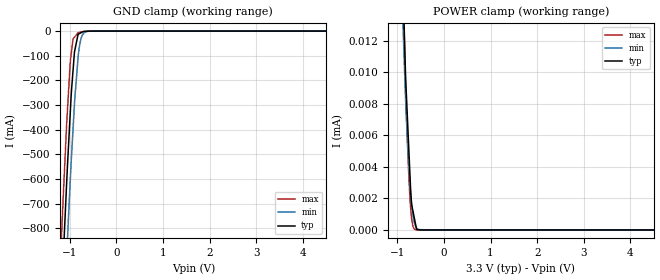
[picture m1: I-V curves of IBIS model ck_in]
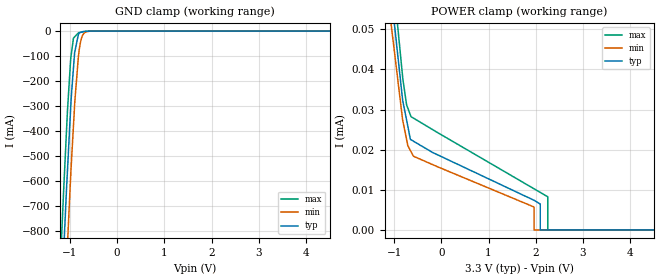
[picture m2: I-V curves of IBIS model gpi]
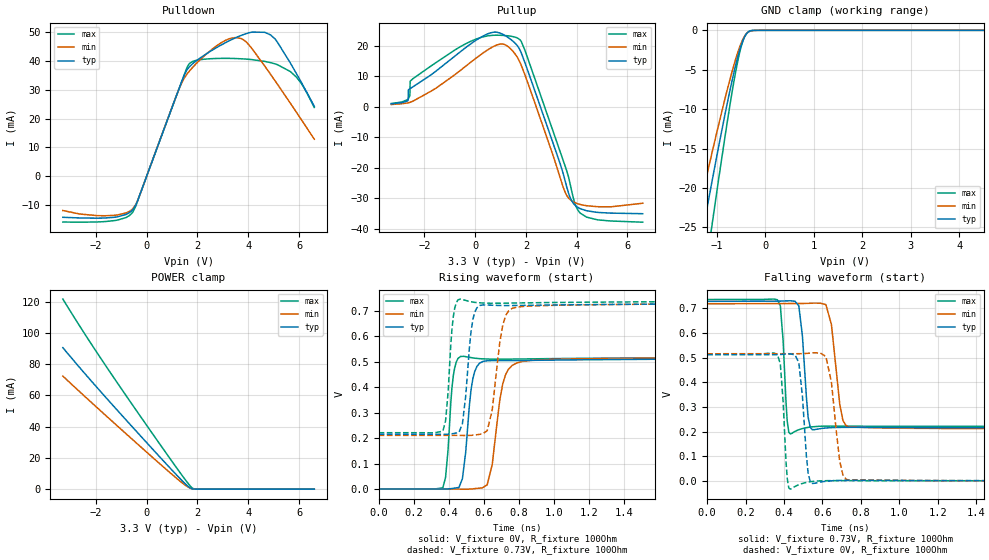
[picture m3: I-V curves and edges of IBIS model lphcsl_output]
|Texas Instruments Incorporated
| Marketing Part # : CDCDB2000
| Voltage Range : 3.3V
| Package-type: TLGA (GQFN)
| #pins/pkg drawing : 80-pin NPP
[IBIS Ver] 3.2
[File name] cdcdb2000.ibs
[File Rev] 1.1
[Date] 04/19/2023
[Source]
| Texas Instruments Incorporated.
| 12500 TI Blvd
| Dallas, TX -75243
[Notes] Revision History:
| Rev 1.1: 04/19/2023
| - Output model updated to take into account impedance values
| - after production trim
| Rev 1.0: 02/18/2019
| - Initial version of the model
| - Model generated from simulations in TISPICE/SPECTRE
| - C_comp although listed in numerical order of value are
| obtained from varying PVT conditions. For PVT conditions for
| each specific value refer the buffer description under
| respective [Model]. IBIS model user is responsible for using
| appropriate C_comp to simulate for Signal Integrity.
| - Warnings regarding combined Non-monotonicity of various models have been
| reviewed and considered minor and can be ignored.
|**** Modify the following if you use [Model Selector]*****************
| - Model names with a trailing _1p8 contain the model for
| 1.8V operation. Model names with a trailing _3p3 contain the model
| for 3.3V operation.
[Disclaimer]
| This model is designed as an aid for customers of Texas Instruments.
| TI and its licensors and suppliers make no warranties, either expressed
| or implied, with respect to this model, including the warranties of
| merchantability or fitness for a particular purpose. The model is
| provided solely on an "as is" basis. The entire risk as to its quality
| and performance is with the customer.
| This model is subject to change without notice. Texas Instruments
| Incorporated is not responsible for updating this model.
[Copyright]
(C) Copyright 2019 Texas Instruments Incorporated. All rights reserved.
| Component1 CDCDB2000 (per package)
[Component] CDCDB2000
[Manufacturer] Texas Instruments Incorporated
[Package] |80 GQFN
| variable typ min max
R_pkg 0.111 0.052 0.169
L_pkg 2.02nH 1.12nH 2.9nH
C_pkg 0.163pF 0.062pF 0.264pF
| pin number (pin name) mapping to model name
[Pin] signal_name model_name R_pin L_pin C_pin
1   DIF_INP   ck_in   NA   NA   NA
2   DIF_INN   ck_in   NA   NA   NA
3   DIF0P   lphcsl_output   NA   NA   NA
4   DIF0N   lphcsl_output   NA   NA   NA
5   DIF1P   lphcsl_output   NA   NA   NA
6   DIF1N   lphcsl_output   NA   NA   NA
7   DIF2P   lphcsl_output   NA   NA   NA
8   DIF2N   lphcsl_output   NA   NA   NA
9   DIF3P   lphcsl_output   NA   NA   NA
10   DIF3N   lphcsl_output   NA   NA   NA
11   DIF4P   lphcsl_output   NA   NA   NA
12   DIF4N   lphcsl_output   NA   NA   NA
13   DIF5P   lphcsl_output   NA   NA   NA
14   DIF5N   lphcsl_output   NA   NA   NA
15   DIF6P   lphcsl_output   NA   NA   NA
16   DIF6N   lphcsl_output   NA   NA   NA
17   DIF7P   lphcsl_output   NA   NA   NA
18   DIF7N   lphcsl_output   NA   NA   NA
19   DIF8P   lphcsl_output   NA   NA   NA
20   DIF8N   lphcsl_output   NA   NA   NA
21   DIF9P   lphcsl_output   NA   NA   NA
22   DIF9N   lphcsl_output   NA   NA   NA
23   DIF10P   lphcsl_output   NA   NA   NA
24   DIF10N   lphcsl_output   NA   NA   NA
25   DIF11P   lphcsl_output   NA   NA   NA
26   DIF11N   lphcsl_output   NA   NA   NA
27   DIF12P   lphcsl_output   NA   NA   NA
28   DIF12N   lphcsl_output   NA   NA   NA
29   DIF13P   lphcsl_output   NA   NA   NA
30   DIF13N   lphcsl_output   NA   NA   NA
31   DIF14P   lphcsl_output   NA   NA   NA
32   DIF14N   lphcsl_output   NA   NA   NA
33   DIF15P   lphcsl_output   NA   NA   NA
34   DIF15N   lphcsl_output   NA   NA   NA
35   DIF16P   lphcsl_output   NA   NA   NA
36   DIF16N   lphcsl_output   NA   NA   NA
37   DIF17P   lphcsl_output   NA   NA   NA
38   DIF17N   lphcsl_output   NA   NA   NA
39   DIF18P   lphcsl_output   NA   NA   NA
40   DIF18N   lphcsl_output   NA   NA   NA
41   DIF19P   lphcsl_output   NA   NA   NA
42   DIF19N   lphcsl_output   NA   NA   NA
43   POWERGD   gpi   NA   NA   NA
44   OE5B/DATA   gpi   NA   NA   NA
45   OE6B/CLK   gpi   NA   NA   NA
46   OE7B   gpi   NA   NA   NA
47   OE8B   gpi   NA   NA   NA
48   OE9B   gpi   NA   NA   NA
49   OE10B/SHIFT_LD   gpi   NA   NA   NA
50   OE11B   gpi   NA   NA   NA
51   OE12B   gpi   NA   NA   NA
52   SADR0   strap_in   NA   NA   NA
53   SADR1   strap_in   NA   NA   NA
54   VDD   POWER   NA   NA   NA
55   SBEN   gpi   NA   NA   NA
56   VDD_A   POWER   NA   NA   NA
57   SMBDAT   smbdat   NA   NA   NA
58   SMBCLK   smbclk   NA   NA   NA
[Diff Pin]   inv_pin   vdiff   tdelay_typ  tdelay_min  tdelay_max
1   2   10m   NA   NA   NA
3   4   NA   NA   NA   NA
5   6   NA   NA   NA   NA
7   8   NA   NA   NA   NA
9   10   NA   NA   NA   NA
11   12   NA   NA   NA   NA
13   14   NA   NA   NA   NA
15   16   NA   NA   NA   NA
17   18   NA   NA   NA   NA
19   20   NA   NA   NA   NA
21   22   NA   NA   NA   NA
23   24   NA   NA   NA   NA
25   26   NA   NA   NA   NA
27   28   NA   NA   NA   NA
29   30   NA   NA   NA   NA
31   32   NA   NA   NA   NA
33   34   NA   NA   NA   NA
35   36   NA   NA   NA   NA
37   38   NA   NA   NA   NA
39   40   NA   NA   NA   NA
41   42   NA   NA   NA   NA
| Use Differential pin definition for differential I/Os
|[Diff Pin] inv_pin vdiff tdelay_typ tdelay_min tdelay_max
|3 4 200mV NA NA NA
|15 16 NA NA NA NA
|***** end of component 1 definition
| Models and submodels in the file (6): ck_in (Input), gpi (Input), lphcsl_output (Output), smbclk (Input), smbdat (I/O_open_drain), strap_in (Input)
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| Model Selectors
|***Modify the following as it applies to a speciic model with multiple ****
|*** powver supply options or driver programmability *********
| Model1
|IBIS Model File - Generated by SIMDE
| http://www.iometh.com/Product/SIMDE
[Model]   ck_in
Model_type   Input
Vinl = 0.66
Vinh = 2.64
|   typ   min   max
C_comp   1.16pF   1.09pF   1.19pF
[Voltage Range]   3.3   3.135   3.465
[Temperature Range]   27   105   -40
[Power Clamp Reference]   3.3   3.135   3.465
[GND Clamp Reference]   0   0   0
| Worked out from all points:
|   GND clamp passes 1 mA (typ) near -0.66 V on its own axis
|   POWER clamp passes 1 mA (typ) near -3.28 V on its own axis
[GND Clamp]
|   Voltage   I(typ)   I(min)   I(max)
-3.3V     -11.22A    -11.44A    -11.05A
-1.173V   -1.062A    -1.366A    -813.7mA
-1.136V   -902.5mA   -1.208A    -656.9mA
-1.079V   -664.6mA   -960.5mA   -423.2mA
-1.053V   -557.2mA   -856mA     -329.6mA
-983.9mV  -310.7mA   -583.3mA   -113.4mA
-930.4mV  -160.9mA   -399.1mA   -32.16mA
-899.2mV  -84.55mA   -294.1mA   -24.93mA
-819.1mV  -12.84mA   -100.7mA   -6.285mA
-733.2mV  -4.01mA    -17.71mA   -3.143mA
-574.9mV  -160.4uA   -530.3uA   -296uA
6.6V      0A         0A         0A
[POWER Clamp]
|   Voltage   I(typ)   I(min)   I(max)
-3.3V     1.02mA     538.7uA    1.487mA
-1.308V   59.88uA    49.8uA     64.78uA
-821.7mV  9.697uA    8.259uA    8.987uA
-767.8mV  6.116uA    4.856uA    4.476uA
-742.7mV  4.452uA    3.567uA    2.814uA
-721.9mV  3.073uA    2.634uA    1.725uA
-711.4mV  2.376uA    2.259uA    1.354uA
-693.3mV  1.637uA    1.625uA    731nA
-636.6mV  790nA      481.6nA    47.81nA
-586.5mV  40.89nA    122.5nA    5.344nA
-503.6mV  0A         20.62nA    0A
6.6V      0A         0A         0A
[Model]   gpi
Model_type   Input
Vinl = 1.2
Vinh = 1.6
|   typ   min   max
C_comp   0.852pF   0.823pF   0.899pF
[Voltage Range]   3.3   3.135   3.465
[Temperature Range]   27   105   -40
[Power Clamp Reference]   3.3   3.135   3.465
[GND Clamp Reference]   0   0   0
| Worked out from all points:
|   GND clamp passes 1 mA (typ) near -0.67 V on its own axis
|   POWER clamp passes 1 mA (typ) near -3.23 V on its own axis
[GND Clamp]
|   Voltage   I(typ)   I(min)   I(max)
-3.3V     -11.22A    -11.44A    -11.05A
-1.169V   -1.043A    -1.347A    -794.9mA
-1.117V   -822.5mA   -1.123A    -578.3mA
-1.052V   -561.1mA   -858mA     -321.1mA
-981.8mV  -301.3mA   -575.6mA   -108.9mA
-924.3mV  -147.1mA   -378.9mA   -28.07mA
-900.2mV  -86.41mA   -297.7mA   -23.27mA
-814.3mV  -11.35mA   -92.89mA   -6.206mA
-776.1mV  -5.231mA   -44.91mA   -4.896mA
-733.4mV  -2.522mA   -17.99mA   -3.434mA
-576.2mV  -234.6uA   -567.7uA   -301.8uA
6.6V      0A         0A         0A
[POWER Clamp]
|   Voltage   I(typ)   I(min)   I(max)
-3.3V     1.056mA    570.2uA    1.534mA
-1.562V   113.2uA    100.1uA    127.7uA
-818.6mV  32.32uA    27.41uA    38.13uA
-594.1mV  22.15uA    18.47uA    27.9uA
1.964V    7.396uA    5.719uA    10.26uA
1.965V    7.392uA    5.625uA    10.26uA
1.965V    7.392uA    0A         10.26uA
2.096V    0A         0A         9.361uA
2.255V    0A         0A         8.268uA
2.255V    0A         0A         8.026uA
2.255V    0A         0A         0A
6.6V      0A         0A         0A
[Model]   lphcsl_output
Model_type   Output
Polarity   Non-Inverting
Vmeas = 0.375
Vref = 0.375
Cref = 2pF
Rref = 100000
|   typ   min   max
C_comp   0.625pF   0.558pF   0.773pF
[Voltage Range]   3.3   3.135   3.465
[Temperature Range]   27   125   -40
[Pullup Reference]   3.3   3.135   3.465
[Pulldown Reference]   -0   -0   -0
[Power Clamp Reference]   3.3   3.135   3.465
[GND Clamp Reference]   0   0   0
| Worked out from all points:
|   slope of the pulldown table from 0 to 0.495 V, typ, clamps not added: 41.7 ohm
|   GND clamp passes 1 mA (typ) near -0.44 V on its own axis
|   falling waveform, V_fixture 0.73V, R_fixture 100Ohm: 20-80 % time 29ps typ, 40.6ps min, 21.3ps max; typ from 0.728 V to 0.215 V
|   rising waveform, V_fixture 0V, R_fixture 100Ohm: 20-80 % time 42.6ps typ, 58.6ps min, 31.4ps max; typ from 0 V to 0.51 V
|   rising waveform, V_fixture 0.73V, R_fixture 100Ohm: 20-80 % time 40ps typ, 54.5ps min, 30.1ps max; typ from 0.215 V to 0.727 V
|   falling waveform, V_fixture 0V, R_fixture 100Ohm: 20-80 % time 29.6ps typ, 43ps min, 22.1ps max; typ from 0.512 V to 0.001 V
[Pulldown]
|   Voltage   I(typ)   I(min)   I(max)
-3.3V     -14.26mA   -11.91mA   -15.9mA
-1.637V   -14.51mA   -13.73mA   -15.74mA
-547.8mV  -11.64mA   -11.28mA   -12.45mA
-260.7mV  -6.256mA   -6.291mA   -6.246mA
1.264V    30.12mA    30.06mA    30.14mA
1.67V     37.85mA    36.36mA    38.96mA
2.65V     44.12mA    44.59mA    40.85mA
3.343V    47.42mA    47.95mA    40.9mA
3.897V    49.43mA    46.82mA    40.67mA
4.877V    49.05mA    35.38mA    39.43mA
5.887V    35.76mA    22.33mA    34.47mA
6.6V      24.26mA    12.85mA    23.87mA
[GND Clamp]
|   Voltage   I(typ)   I(min)   I(max)
-3.3V     -95.21mA   -78.35mA   -123.7mA
-1.538V   -33.84mA   -27.44mA   -43.92mA
-1.34V    -27.13mA   -21.99mA   -35.15mA
-1.241V   -23.81mA   -19.3mA    -30.8mA
-1.112V   -19.56mA   -15.85mA   -25.22mA
-1.003V   -16.02mA   -12.99mA   -20.56mA
-815.1mV  -10.12mA   -8.246mA   -12.78mA
-587.4mV  -3.811mA   -3.16mA    -4.469mA
-458.7mV  -1.229mA   -1.073mA   -1.272mA
-389.4mV  -433.8uA   -414.9uA   -415uA
-320.1mV  -93.44uA   -113.8uA   -78.75uA
6.6V      0A         0A         0A
[Pullup]
|   Voltage   I(typ)   I(min)   I(max)
-3.3V     954.3uA    732.8uA    1.056mA
-2.637V   2.12mA     1.291mA    2.559mA
-2.627V   5.549mA    1.309mA    2.656mA
-2.567V   5.892mA    1.44mA     3.69mA
-2.558V   5.947mA    1.466mA    8.374mA
-2.449V   6.527mA    1.821mA    9.191mA
432.3mV   23.67mA    18.3mA     23.14mA
1.125V    23.59mA    20.53mA    23.38mA
1.68V     19.83mA    15.99mA    22.47mA
3.551V    -24.51mA   -28.15mA   -19.62mA
4.046V    -33.01mA   -31.84mA   -33.9mA
6.6V      -35.08mA   -31.64mA   -37.86mA
[POWER Clamp]
|   Voltage   I(typ)   I(min)   I(max)
-3.3V     90.61mA    72.41mA    121.7mA
-2.162V   68.92mA    55.3mA     92.49mA
-815.1mV  44.38mA    35.53mA    60mA
1.214V    8.474mA    6.479mA    12.85mA
1.61V     2.102mA    1.548mA    4.142mA
1.798V    256.2uA    261uA      767.7uA
1.967V    5.611uA    12.37uA    12.29uA
6.6V      0A         0A         0A
[Ramp]
R_load = 100
|   typ   min   max
dV/dt_r   0.305979/4.26211e-11   0.308993/5.85849e-11   0.309345/3.13767e-11
dV/dt_f   0.307804/2.8961e-11   0.30405/4.06149e-11   0.308924/2.13477e-11
[Falling Waveform]
V_fixture = 0.73V
V_fixture_min = 0.72V
V_fixture_max = 0.75V
R_fixture = 100Ohm
C_fixture = 0F
|   Time   V(typ)   V(min)   V(max)
0s        728.4mV    718.5mV    735.8mV
365.6ps   729.1mV    719.4mV    735mV
380.9ps   729.4mV    719.4mV    710.4mV
432.6ps   730.8mV    719.5mV    190.5mV
477.1ps   710.5mV    719.6mV    207.3mV
525.7ps   257mV      720.3mV    216.9mV
546.8ps   207.7mV    721mV      219.3mV
646.9ps   215.7mV    633.8mV    222.1mV
723.8ps   217.1mV    222.7mV    221.9mV
2ns       215.4mV    211.8mV    220.9mV
[Rising Waveform]
V_fixture = 0V
V_fixture_min = 0V
V_fixture_max = 0V
R_fixture = 100Ohm
C_fixture = 0F
|   Time   V(typ)   V(min)   V(max)
0s        440.1uV    71.87nV    -287.1nV
365.6ps   77.71uV    -55.3uV    5.352mV
424.9ps   2.977mV    -92.83uV   443.7mV
467.2ps   23.53mV    -300.3uV   520.2mV
536.7ps   433.8mV    870.7uV    514.2mV
595.7ps   500.9mV    6.928mV    510.6mV
646.9ps   503.8mV    96.35mV    509.5mV
706.6ps   503.9mV    412mV      509.5mV
788.2ps   504.1mV    494.9mV    510mV
2ns       510.4mV    515mV      515.6mV
[Rising Waveform]
V_fixture = 0.73V
V_fixture_min = 0.72V
V_fixture_max = 0.75V
R_fixture = 100Ohm
C_fixture = 0F
|   Time   V(typ)   V(min)   V(max)
0s        215mV      210.6mV    220.9mV
365.6ps   214.6mV    210.5mV    227.4mV
452.1ps   221.3mV    210.4mV    742.1mV
477.1ps   256.3mV    210.2mV    743.3mV
536.7ps   665.4mV    211.3mV    733.2mV
575.3ps   719.8mV    214.7mV    730.5mV
618.1ps   721.7mV    228.4mV    729.1mV
706.6ps   719.8mV    642.2mV    728.9mV
760.3ps   719.8mV    708.4mV    729.4mV
2ns       726.8mV    727mV      735.8mV
[Falling Waveform]
|Gnd
V_fixture = 0V
V_fixture_min = 0V
V_fixture_max = 0V
R_fixture = 100Ohm
C_fixture = 0F
|   Time   V(typ)   V(min)   V(max)
0s        511.5mV    515mV      515.6mV
365.6ps   512.2mV    515.8mV    512.7mV
380.9ps   512.7mV    515.8mV    474mV
432.6ps   515.5mV    515.9mV    -33.87mV
477.1ps   480mV      515.9mV    -15.8mV
525.7ps   29.97mV    517.7mV    -5.351mV
546.8ps   -10.63mV   519.2mV    -2.694mV
618.1ps   -1.882mV   504.3mV    473.8uV
723.8ps   1.96mV     5.711mV    775.4uV
2ns       591.7uV    71.87nV    -287.1nV
